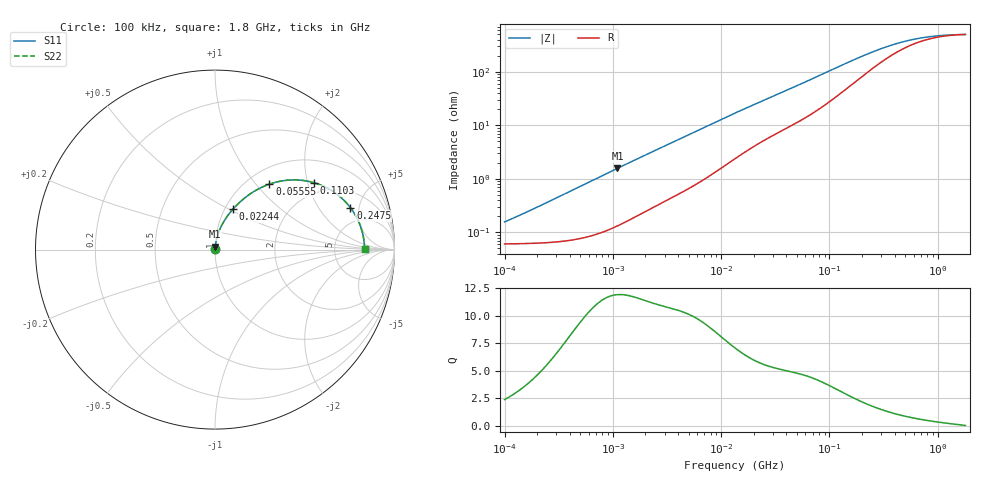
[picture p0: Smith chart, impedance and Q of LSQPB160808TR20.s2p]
! LSQPB160808TR20  S-PARAMETER MODEL  ( General Type )
! Model Generated by TAIYO YUDEN Corporation (http://www.ty-top.com)
! Version 5.0
! TAIYO YUDEN Control No. 110926NF18SB-HKC
! Copyright(c) 2007 TAIYO YUDEN CO.,LTD. All Rights Reserved.
! Product Description (link to TY-COMPAS)
! https://ds.yuden.co.jp/TYCOMPAS/or/detail?pn=LSQPB160808TR20M&u=M
! Products Name : Inductors
! Characteristics :
!  Inductance : 0.20 uH , SRF(min) : 400 MHz , DC Resistance(max) : 0.078 Ohm
!  Rated Current : Saturation :1750 mA , Temp Rise : 980 mA (40 degC)
!  Case Size : 1.6 x 0.8 / 0.063 x 0.031 [mm/inch] , Thickness : 0.8 / 0.031 [mm/inch]
!  (Conditions: Temperature = 25 degC , DC Bias Current/Voltage = 0A / 0V)
! External Node Assignments :
!  1  o---GGG---o  2
! GND o---------o GND
! Frequency Range : 0.1MHz  -  1800MHz  [ 402 STEP ]
# MHz S RI R 50
! Freq[MHz].  S11 Real  S11 Imag  S21 Real  S21 Imag  S12 Real  S12 Imag  S22 Real  S22 Imag
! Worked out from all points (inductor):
!   401 points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, 100 kHz to 1.8 GHz, reference 50 ohm
!   read as one part in series: L = 230 nH near 127.8 kHz
!   highest Q = 11.9 at 1.103 MHz (marker M1), where L = 226 nH
!   S11 on the Smith chart (normalised r, x): 100 kHz: 1.00, +0.00; 22.44 MHz: 1.09, +0.53; 55.55 MHz: 1.25, +1.18; 110.3 MHz: 1.64, +2.19; 247.5 MHz: 3.28, +4.07; 1.8 GHz: 11, +0
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0.1  0.000609 0.00144  0.9994 -0.00144  0.9994 -0.00144  0.000609 0.00144
0.113029  0.000611 0.00163  0.9994 -0.00163  0.9994 -0.00163  0.000611 0.00163
0.171412  0.000626 0.00247  0.9994 -0.00247  0.9994 -0.00247  0.000626 0.00247
0.516129  0.00083 0.00742  0.9992 -0.00742  0.9992 -0.00742  0.00083 0.00742
1.102914  0.00156 0.0156  0.9984 -0.0156  0.9984 -0.0156  0.00156 0.0156
2.66389  0.00463 0.0362  0.9954 -0.0362  0.9954 -0.0362  0.00463 0.0362
6.278453  0.0151 0.0804  0.9849 -0.0804  0.9849 -0.0804  0.0151 0.0804
13.41641  0.0487 0.1557  0.9513 -0.1557  0.9513 -0.1557  0.0487 0.1557
22.44079  0.1018 0.2275  0.8982 -0.2275  0.8982 -0.2275  0.1018 0.2275
35.74074  0.1836 0.3015  0.8164 -0.3015  0.8164 -0.3015  0.1836 0.3015
44.5561  0.2378 0.3358  0.7622 -0.3358  0.7622 -0.3358  0.2378 0.3358
55.54574  0.3035 0.3649  0.6965 -0.3649  0.6965 -0.3649  0.3035 0.3649
69.24595  0.3796 0.3838  0.6204 -0.3838  0.6204 -0.3838  0.3796 0.3838
86.32529  0.4617 0.3878  0.5383 -0.3878  0.5383 -0.3878  0.4617 0.3878
110.2859  0.5518 0.3726  0.4482 -0.3726  0.4482 -0.3726  0.5518 0.3726
167.2511  0.6786 0.3093  0.3214 -0.3093  0.3214 -0.3093  0.6786 0.3093
247.5026  0.7548 0.2332  0.2452 -0.2332  0.2452 -0.2332  0.7548 0.2332
357.3983  0.7947 0.1679  0.2053 -0.1679  0.2053 -0.1679  0.7947 0.1679
528.8877  0.8165 0.112  0.1835 -0.112  0.1835 -0.112  0.8165 0.112
763.7235  0.8264 0.0717  0.1736 -0.0717  0.1736 -0.0717  0.8264 0.0717
1158.204  0.8315 0.0362  0.1685 -0.0362  0.1685 -0.0362  0.8315 0.0362
1800  0.8332 0.00497  0.1668 -0.00497  0.1668 -0.00497  0.8332 0.00497
